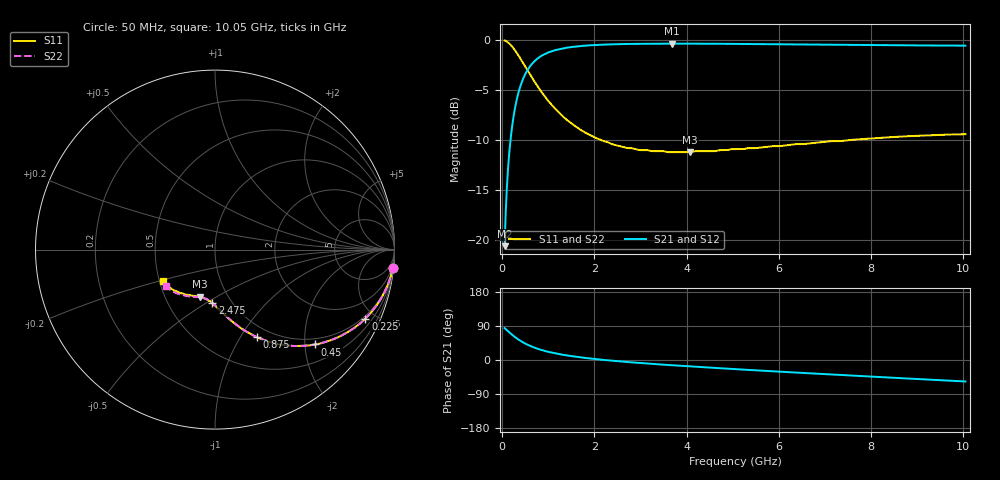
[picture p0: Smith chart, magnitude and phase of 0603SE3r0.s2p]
! AVX Thin Film Operation		Date: August 2001
! Description: Accu-P® Series, Thin Film, SMD, RF Capacitor
! Part Number: 06035J3R0ABT
! 50 MHz  -  10.05 GHz
! Serial Measurements
# mhz S db R 50
!	S11		S21		S12		S22
!	dB	Phase	dB	Phase	dB	Phase	dB	Phase
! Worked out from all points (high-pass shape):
!   401 points, 50 MHz to 10.05 GHz, reference 50 ohm
!   highest |S21| = -0.36 dB at 3.675 GHz (marker M1); lowest = -20.6 dB at 50 MHz (marker M2)
!   |S21| within 3 dB of the highest: 502.8 MHz to end of sweep
!   lowest |S11| = -11.2 dB at 4.075 GHz (marker M3), VSWR 1.76, Z = 37.2 - j21.1 ohm
!   |S11| at or under -10 dB: 2.147 GHz to 7.514 GHz (5.367 GHz wide, 111 % of centre)
!   |S22| runs from -11.2 to 0.0 dB; largest |S21 - S12| = 0
!   S11 on the Smith chart (normalised r, x): 50 MHz: 1, -20; 225 MHz: 0.87, -4.42; 450 MHz: 0.86, -2.23; 875 MHz: 0.86, -1.18; 2.475 GHz: 0.81, -0.53; 10.05 GHz: 0.52, -0.21
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50  -0.04 -5.8  -20.60 84.2  -20.60 84.2  -0.04 -5.8
75  -0.09 -8.6  -17.11 81.4  -17.11 81.4  -0.09 -8.6
125  -0.23 -14.3  -12.79 75.7  -12.79 75.7  -0.23 -14.3
150  -0.33 -17.0  -11.32 73.0  -11.32 73.0  -0.33 -17.0
175  -0.44 -19.5  -10.15 70.5  -10.15 70.5  -0.44 -19.5
225  -0.71 -24.6  -8.24 65.4  -8.24 65.4  -0.71 -24.6
325  -1.36 -33.8  -5.72 56.1  -5.72 56.1  -1.36 -33.8
450  -2.29 -43.5  -3.88 46.5  -3.88 46.5  -2.29 -43.5
550  -3.05 -49.8  -2.97 40.2  -2.97 40.2  -3.05 -49.8
650  -3.80 -55.1  -2.35 34.9  -2.35 34.9  -3.80 -55.1
875  -5.34 -64.4  -1.51 25.6  -1.51 25.6  -5.34 -64.3
1050  -6.34 -69.8  -1.16 20.2  -1.16 20.2  -6.34 -69.8
1250  -7.33 -74.7  -0.89 15.2  -0.89 15.2  -7.33 -74.6
1725  -9.04 -83.5  -0.58 6.5  -0.58 6.5  -9.04 -83.2
2475  -10.52 -93.0  -0.41 -2.9  -0.41 -2.9  -10.52 -92.5
3400  -11.10 -101.8  -0.36 -11.5  -0.36 -11.5  -11.10 -100.8
3675  -11.20 -103.9  -0.36 -13.8  -0.36 -13.8  -11.19 -102.9
4075  -11.20 -107.6  -0.36 -16.9  -0.36 -16.9  -11.14 -106.0
5050  -10.90 -114.8  -0.38 -24.1  -0.38 -24.1  -10.90 -112.8
6725  -10.30 -127.0  -0.45 -35.4  -0.45 -35.4  -10.30 -123.0
8400  -9.71 -138.2  -0.51 -46.3  -0.51 -46.3  -9.68 -134.1
10050  -9.41 -148.8  -0.56 -56.6  -0.56 -56.6  -9.37 -143.6
